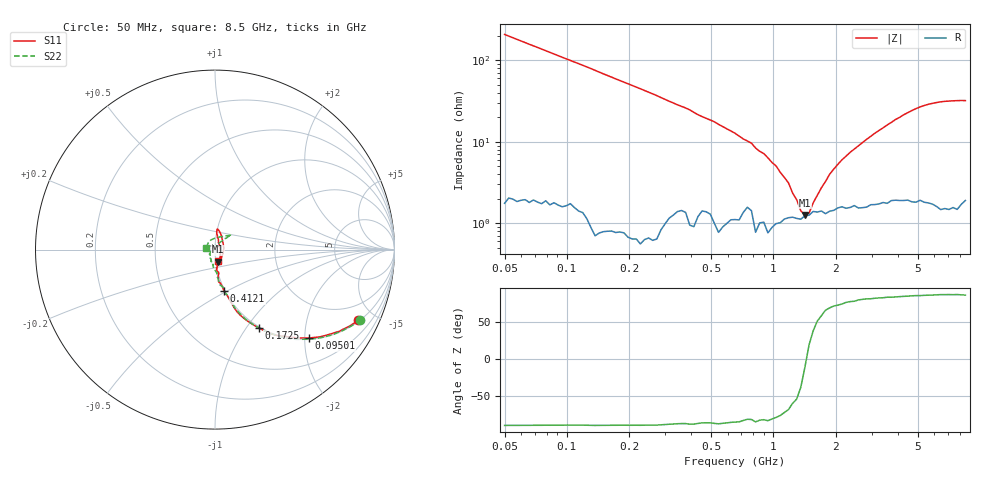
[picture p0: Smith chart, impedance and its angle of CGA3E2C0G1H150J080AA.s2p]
! S-parameter Generated by TDK Corporation
! Copyright(C) 2015 TDK Corporation.
! All Rights Reserved.
! TDK P/N: CGA3E2C0G1H150J080AA (Multilayer Ceramic Chip Capacitors)
! Property: C=15pF
! Size(LxWxT): 1.6x0.8x0.8mm, 0.063x0.031x0.031inches
! Model Type: s2p (Touchstone File Format Version 1.0)
! Frequency: DC=Yes Start=50MHz Stop=8500MHz 114points Log-sweep
! Note:
! Model Generated on Jun. 23, 2015
! Hash(MD5):
! Port Assignments:
!  1 ---| |--- 2
! Applicable Conditions:
!  Temperature = 25 degC
!  DC Bias Voltage = 0 V
!  Small Signal Operation
! Terms and conditions regarding TDK Simulation Models
! (1)This simulation model is being provided solely for informational purposes. Please refer to the specifications of the products in terms of detailed characteristics of such products.
! (2)In no event shall TDK Corporation of any of its subsidiaries be liable for any loss or damage arising, directly or indirectly,
!  From any information contained in this simulation model, including, but not limited to loss or damages arising from any inaccuracies, omissions or errors in connection with such information.
! (3)Any and all copyrights on this simulation model are owned by TDK Corporation.
!  Duplication or redistribution of this simulation model without prior written permission from TDK Corporation is prohibited.
! (4)This simulation model is subject to any modification or change without any prior notice.
! (5)Neither TDK Corporation nor any of its subsidiaries shall make any warranty, express or implied,
!  Including but not limited to the correctness, implied warranties of merchantability and fitness for a particular purpose with respect to this simulation models.
! (6)The use of this simulation model shall be deemed to have consented to the terms and conditions hereof.
# MHz S MA R 50
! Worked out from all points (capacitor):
!   113 points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, 50 MHz to 8.5 GHz, reference 50 ohm
!   read as one part in series: C = 15.4 pF near 50 MHz
!   lowest |Z| = 1.27 ohm at 1.421 GHz (marker M1)
!   series resonance near 1.445 GHz, so ESL is about 790 pH
!   S11 on the Smith chart (normalised r, x): 50 MHz: 1.06, -4.00; 95.01 MHz: 1.03, -2.09; 172.5 MHz: 0.98, -1.14; 412.1 MHz: 0.99, -0.49; 8.5 GHz: 1.03, -0.13
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50  0.8893 -26.4  0.432 63.4  0.4322 63.4  0.898 -25.9
95.01149  0.7173 -43.4  0.6646 46.5  0.6641 46.5  0.7353 -42.5
119.495  0.6364 -49.8  0.7405 40.0  0.7402 40.0  0.6556 -49.3
172.4517  0.499 -60.9  0.8436 29.8  0.8433 29.8  0.5159 -59.6
285.5811  0.3405 -71.8  0.9254 18.2  0.9252 18.3  0.3314 -71.7
412.1423  0.2383 -77.6  0.9567 11.6  0.9581 11.6  0.2377 -77.1
651.9202  0.1566 -83.3  0.9672 5.3  0.9663 5.4  0.1506 -85.6
1421.493  0.06945 -76.0  0.9753 -3.7  0.9735 -3.6  0.06855 -109.0
1558.024  0.06537 -71.3  0.9737 -4.8  0.9746 -4.7  0.05994 -112.5
2354.001  0.04007 -42.9  0.9722 -9.8  0.9724 -9.8  0.03652 -142.5
2827.91  0.02772 -10.6  0.9722 -12.5  0.9721 -12.5  0.02081 -169.6
3099.524  0.02966 21.8  0.9712 -13.9  0.9705 -13.9  0.01456 143.3
3244.963  0.02806 37.1  0.9704 -14.7  0.9691 -14.7  0.01594 103.4
3397.226  0.03516 44.9  0.9704 -15.5  0.9704 -15.6  0.02007 83.6
3723.522  0.04873 66.4  0.9677 -17.3  0.9684 -17.3  0.04096 59.0
4272.658  0.08193 80.9  0.9639 -20.1  0.964 -20.2  0.07931 49.0
4683.036  0.09973 84.6  0.9624 -22.4  0.9613 -22.3  0.1029 44.8
5373.679  0.116 83.1  0.9587 -25.8  0.9582 -25.8  0.122 41.5
6166.175  0.1004 74.2  0.9571 -29.8  0.9584 -29.7  0.1072 46.8
7407.553  0.05 8.7  0.9593 -36.1  0.9589 -36.1  0.06305 91.2
7755.137  0.04898 -23.8  0.9589 -38.0  0.9584 -37.9  0.05846 113.6
8500  0.06431 -72.6  0.9548 -42.0  0.9546 -41.7  0.05018 169.0
